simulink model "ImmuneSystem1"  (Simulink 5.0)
settings: Solver=ode45  StartTime=0.0  StopTime=10.0  RelTol=1e-3
undefined symbols (not defined in the file or in its folder): sigbuilder_block

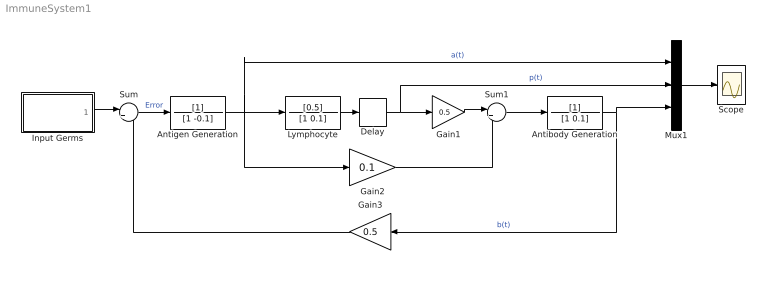
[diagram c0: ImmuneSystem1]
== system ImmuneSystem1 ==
  Antibody Generation : TransferFcn  Denominator=[1 0.1]
  Antigen Generation : TransferFcn  Denominator=[1 -0.1]
  Delay : TransportDelay  DelayTime=0.2
  Gain1 : Gain  Gain=0.5
  Gain2 : Gain  Gain=0.1
  Gain3 : Gain  Orientation=left  Gain=0.5
  Input Germs : Subsystem  Tag=STV Subsys  StartFcn=sigbuilder_block('start');  StopFcn=sigbuilder_block('stop');  ClipboardFcn=sigbuilder_block('clipboard');
  Lymphocyte : TransferFcn  Numerator=[0.5]  Denominator=[1 0.1]
  Mux1 : Mux  Inputs=3
  Scope : Scope
  Sum : Sum  Inputs=|+-
  Sum1 : Sum  Inputs=|+-
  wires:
  Input Germs/1(Germs) -> Sum/1
  Gain3/1 -> Sum/2
  Lymphocyte/1 -> Delay/1
  Gain1/1 -> Sum1/1
  Sum1/1 -> Antibody Generation/1
  Gain2/1 -> Sum1/2
  Antigen Generation/1 -> Gain2/1, Lymphocyte/1, Mux1/1  "a(t)"
  Sum/1 -> Antigen Generation/1  "Error"
  Antibody Generation/1 -> Gain3/1, Mux1/3  "b(t)"
  Delay/1 -> Gain1/1, Mux1/2  "p(t)"
  Mux1/1 -> Scope/1

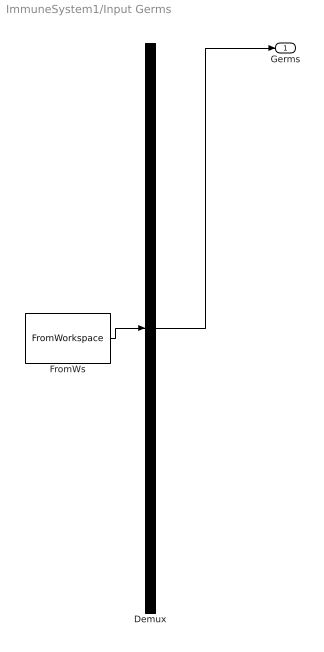
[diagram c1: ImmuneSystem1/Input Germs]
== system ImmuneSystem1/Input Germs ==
  Demux : Demux  Tag=STV Demux  Outputs=1
  FromWs : FromWorkspace  Tag=STV FromWs  VariableName=tuvar  SampleTime=0  SigBuilderData=DataTag0
  Germs : Outport  Tag=STV Outport
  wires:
  Demux/1 -> Germs/1
  FromWs/1 -> Demux/1
